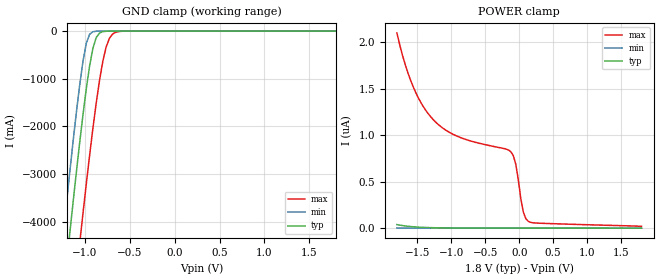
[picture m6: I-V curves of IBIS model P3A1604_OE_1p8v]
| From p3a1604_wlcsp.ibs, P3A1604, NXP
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[Model] P3A1604_OE_1p8v
Model_type Input
Polarity   Non-Inverting
Enable   Active-High
Vinl =  0.734V
Vinh =  0.901V
C_comp   2.027pF   1.667pF   2.300pF
[Model Spec]
Vinh   0.901V   0.751V   1.075V
Vinl   0.734V   0.615V   0.858V
[Temperature Range]   27.000   -40.000   125
[Voltage Range]   1.800V   1.620V   1.980V
[POWER Clamp Reference]   1.800V   1.620V   1.980V
[GND Clamp Reference]   0.0V   0.0V   0.0V
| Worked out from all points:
|   GND clamp passes 1 mA (typ) near -0.70 V on its own axis
[GND_clamp]
|Voltage   I(typ)   I(min)   I(max)
-1.8V     -16.15A    -14.91A    -18.3A
-1.245V   -5.602A    -4.307A    -7.782A
-1.171V   -4.263A    -2.976A    -6.433A
-1.06V    -2.351A    -1.141A    -4.463A
-1.023V   -1.761A    -636.4mA   -3.829A
-986mV    -1.213A    -258.9mA   -3.21A
-912mV    -361.3mA   -13mA      -2.041A
-838mV    -39.5mA    -1.179mA   -1.03A
-764mV    -3.283mA   -693.8uA   -331mA
-727mV    -1.393mA   -597.8uA   -147.6mA
-653mV    -665uA     -423.9uA   -21.28mA
1.8V      0A         0A         0A
[POWER_clamp]
|Voltage   I(typ)   I(min)   I(max)
-1.8V     38.5nA     1.499nA    2.101uA
-1.678V   24.08nA    992pA      1.762uA
-1.567V   15.52nA    720.5pA    1.534uA
-1.419V   8.602nA    522.7pA    1.317uA
-1.271V   4.887nA    425.9pA    1.173uA
-901mV    1.81nA     326pA      986nA
-124mV    1.136nA    209.7pA    823.6nA
-50mV     1.003nA    185pA      688nA
24mV      460.4pA    50.8pA     317nA
61mV      280.3pA    15.75pA    172.4nA
135mV     199.3pA    6.668pA    72.8nA
1.8V      0A         0A         19.22nA
